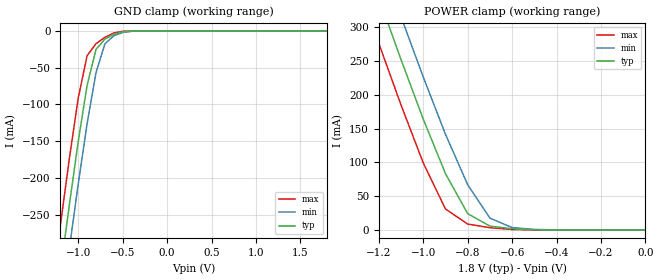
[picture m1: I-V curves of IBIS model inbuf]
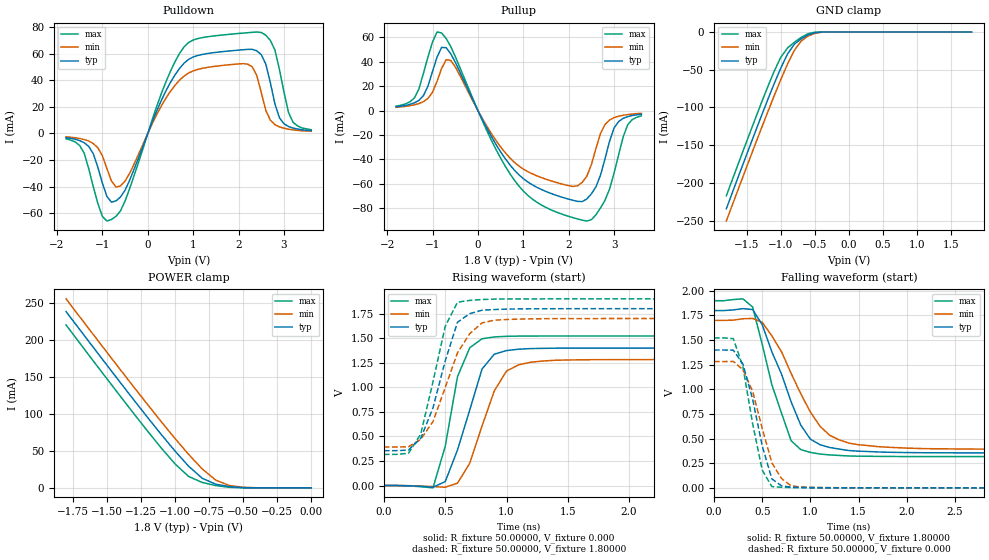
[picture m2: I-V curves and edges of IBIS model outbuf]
| IBIS file ics651_1p8.ibs created by s2ibis2 version 1.2
| North Carolina State University Electronics Research Laboratory  1995
[IBIS ver]   3.2
[File name]   ics651_1p8.ibs
[File Rev]   1.0
[Date]   March 22, 2007
[Source]   IDT
[Notes]   1. Temp typ=25C, min=+85C, max=-40C 2. Ramp rates based on 50
   ohm load
[Disclaimer] READ THESE TERMS AND CONDITIONS CAREFULLY BEFORE USING THIS
   IBIS MODEL. BY USING THIS IBIS MODEL, YOU ARE ACCEPTING AND
   AGREEING TO THESE TERMS AND CONDITIONS OF USE. Integrated
   Device Technology, Inc. ("IDT") hereby grants the user of this
   IBIS model ("User") a non-exclusive, nontransferable license
   to use this IBIS model under the following terms: The User is
   granted this license only to use the IBIS model for
   demonstration purposes only and is not granted rights to sell,
   copy (except as needed to run the IBIS model), rent, lease or
   sub-license (except for demonstration) the IBIS model in whole
   or in part, or in modified form to anyone. The User may modify
   the IBIS model to suit its specific applications, but rights
   to derivative works and such modifications shall belong to
   IDT. THIS IBIS MODEL IS PROVIDED ON AN AS IS" BASIS AND IDT
   MAKES ABSOLUTELY NO WARRANTY WITH RESPECT TO THE INFORMATION
   CONTAINED HEREIN. IDT DISCLAIMS AND USER WAIVES ALL
   WARRANTIES, EXPRESS AND IMPLIED, INCLUDING WARRANTIES OF
   MERCHANTABILITY AND FITNESS FOR A PARTICULAR PURPOSE. THE
   ENTIRE RISK AS TO QUALITY AND PERFORMANCE IS WITH THE USER
   ACCORDINGLY, IN NO EVENT SHALL IDT BE LIABLE FOR ANY DIRECT OR
   INDIRECT DAMAGES, WHETHER IN CONTRACT OR TORT, INCLUDING ANY
   LOST PROFITS OR OTHER INCIDENTAL, CONSEQUENTIAL, EXEMPLARY, OR
   PUNITIVE DAMAGES ARISING OUT OF THE USE OR APPLICATION OF THE
   IBIS MODEL, WHETHER OR NOT IDT HAD NOTICE OF SUCH DAMAGES. IDT
   reserves the right to make changes without notice to any
   product herein to improve reliability, function, or design.
   IDT does not convey any license under patent rights or any
   other intellectual property rights, including those of third
   parties. IDT is not obligated to provide maintenance or
   support for the licensed IBIS model.
   **************************************** This model is for
   ICS651 IDT Clock ****************************************
[Copyright]   Copyright 2007, Integrated Device Technology, Inc. All rights
   reserved.
|   Component ICS651
[Component]   ICS651
[Manufacturer]   Integrated Device Technology Inc.
[Package]
| variable   typ   min   max
R_pkg   40.00000m   35.00000m   45.00000m
L_pkg   1.65000nH   1.35000nH   1.95000nH
C_pkg   0.24000pF   0.14000pF   0.34000pF
[Pin]  signal_name   model_name   R_pin   L_pin   C_pin
1   ICLK   inbuf
2   Q1   outbuf
3   Q2   outbuf
4   Q3   outbuf
5   Q4   outbuf
6   GND   GND
7   VDD   POWER
8   OE   inbuf
| Models and submodels in the file (2): inbuf (Input), outbuf (3-state)
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| in   in   dummy
| oe   oe   dummy
|   Model inbuf
[Model]   inbuf
Model_type   Input
Vinl =  0.63000V
Vinh =  1.17000V
C_comp   5.50000pF   5.00000pF   6.00000pF
[Temperature Range]   25.00000   85.00000   -40.00000
[Voltage Range]   1.80000V   1.70000V   1.90000V
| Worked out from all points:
|   GND clamp passes 1 mA (typ) near -0.50 V on its own axis
|   POWER clamp passes 1 mA (typ) near -0.55 V on its own axis
[GND_clamp]
| voltage   I(typ)   I(min)   I(max)
-1.8V     -898.9mA   -957.2mA   -837.5mA
-1.3V     -420.5mA   -480.4mA   -357mA
-1.2V     -327.6mA   -387.6mA   -264mA
-1.1V     -237mA     -296.6mA   -174mA
-1V       -150.5mA   -208.5mA   -91.29mA
-900mV    -73.81mA   -126.1mA   -33.43mA
-800mV    -24.96mA   -56.58mA   -17.15mA
-700mV    -10.96mA   -17.4mA    -8.598mA
-600mV    -4.471mA   -6.338mA   -2.511mA
-500mV    -925.8uA   -1.904mA   -242.1uA
-400mV    -81.45uA   -291.4uA   -13.93uA
1.8V      1.081nA    848.9nA    -1.089uA
[POWER_clamp]
| voltage   I(typ)   I(min)   I(max)
-1.8V     917.2mA    979.2mA    852mA
-1.3V     437.3mA    500.8mA    369.9mA
-1.2V     343.8mA    407.4mA    276.2mA
-1.1V     252.2mA    315.6mA    185mA
-1V       164.1mA    226.4mA    99.28mA
-900mV    83.43mA    141.7mA    31.04mA
-800mV    24.16mA    66.96mA    8.749mA
-700mV    5.751mA    17.53mA    3.41mA
-600mV    1.751mA    3.532mA    720.7uA
-500mV    298.4uA    782.1uA    64.85uA
-400mV    30.44uA    115.8uA    7.502uA
0V        1.081nA    29.2nA     102.5pA
|   Model outbuf
[Model]   outbuf
Model_type   3-state
Polarity   Non-Inverting
Enable   Active-Low
Vmeas =  0.90000V
Rref = 50.00000
Vref =  0.000V
C_comp   5.50000pF   5.00000pF   6.00000pF
[Temperature Range]   25.00000   85.00000   -40.00000
[Voltage Range]   1.80000V   1.70000V   1.90000V
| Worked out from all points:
|   slope of the pulldown table from 0 to 0.27 V, typ, clamps not added: 11.9 ohm
|   slope of the pullup table from 0 to 0.27 V, typ, clamps not added: 13.8 ohm
|   GND clamp passes 1 mA (typ) near -0.50 V on its own axis
|   POWER clamp passes 1 mA (typ) near -0.55 V on its own axis
|   rising waveform, R_fixture 50.00000, V_fixture 0.000: 20-80 % time 210ps typ, 223ps min, 160ps max; typ from 0 V to 1.4 V
|   rising waveform, R_fixture 50.00000, V_fixture 1.80000: 20-80 % time 209ps typ, 244ps min, 173ps max; typ from 0.355 V to 1.8 V
|   falling waveform, R_fixture 50.00000, V_fixture 1.80000: 20-80 % time 344ps typ, 415ps min, 278ps max; typ from 1.8 V to 0.355 V
|   falling waveform, R_fixture 50.00000, V_fixture 0.000: 20-80 % time 205ps typ, 219ps min, 172ps max; typ from 1.4 V to 0 V
[Pulldown]
| voltage   I(typ)   I(min)   I(max)
-1.8V     -3.2mA     -2.5mA     -4mA
-1.3V     -9.8mA     -5.7mA     -26.65mA
-1V       -37.38mA   -16.83mA   -62.43mA
-800mV    -51.67mA   -35.82mA   -64.64mA
-500mV    -42.63mA   -35.75mA   -50.75mA
300mV     24.94mA    20.82mA    30.1mA
800mV     52.83mA    43.14mA    65.09mA
2.4V      62.08mA    43.6mA     76.17mA
2.6V      52.01mA    17.3mA     73.75mA
2.9V      11.67mA    4.9mA      48mA
3.2V      4mA        2.7mA      8.35mA
3.6V      2.1mA      1.7mA      2.8mA
[Pullup]
| voltage   I(typ)   I(min)   I(max)
-1.8V     3.1mA      2.6mA      3.6mA
-1.4V     6.3mA      4.7mA      10.3mA
-1.2V     12.23mA    7.3mA      30.55mA
-800mV    51.83mA    34.56mA    63.73mA
-600mV    46.63mA    41.18mA    52.66mA
900mV     -52.67mA   -45.5mA    -61.86mA
2.1V      -73.75mA   -62.33mA   -88mA
2.4V      -72.54mA   -53.8mA    -90.69mA
2.8V      -39.53mA   -11.4mA    -73.56mA
3V        -14.21mA   -5.8mA     -51.09mA
3.3V      -5mA       -3.3mA     -11.6mA
3.6V      -3mA       -2.3mA     -4.3mA
[GND_clamp]
| voltage   I(typ)   I(min)   I(max)
-1.8V     -234.3mA   -250.6mA   -217.2mA
-1.3V     -114.7mA   -131.2mA   -97.35mA
-1.1V     -69.05mA   -85.13mA   -52.51mA
-1V       -47.67mA   -63.05mA   -33.38mA
-900mV    -28.89mA   -42.27mA   -21.03mA
-800mV    -16.04mA   -24.21mA   -13.46mA
-700mV    -8.94mA    -11.82mA   -7.05mA
-600mV    -3.886mA   -5.387mA   -2.229mA
-500mV    -872.3uA   -1.753mA   -231uA
-400mV    -76.24uA   -282.3uA   -7.635uA
1.8V      1.081nA    92.98nA    85.97pA
[POWER_clamp]
| voltage   I(typ)   I(min)   I(max)
-1.8V     238.4mA    255.6mA    220.3mA
-1.4V     142mA      159.4mA    123.5mA
-1.2V     94.87mA    112.3mA    76.35mA
-1V       49.75mA    66.73mA    32.37mA
-900mV    29.23mA    45.17mA    15.35mA
-800mV    12.89mA    25.5mA     7.266mA
-700mV    4.877mA    10.33mA    3.05mA
-600mV    1.627mA    3.084mA    683.2uA
-500mV    287.7uA    748.1uA    58.05uA
-400mV    26.31uA    111.6uA    2.376uA
0V        1.081nA    29.2nA     102.5pA
[Ramp]
| variable   typ   min   max
dV/dt_r   0.83940/0.17056n   0.76920/0.21229n   0.91320/0.13298n
dV/dt_f   0.86700/0.31530n   0.78468/0.40017n   0.94968/0.24247n
R_load = 50.00000
[Rising Waveform]
R_fixture = 50.00000
V_fixture = 0.000
V_fixture_min = 0.000
V_fixture_max = 0.000
| time   V(typ)   V(min)   V(max)
0s        0V         0V         0V
400ps     -16.88mV   -10.28mV   -23.47mV
500ps     40.1mV     -17.2mV    399.2mV
600ps     362mV      23.92mV    1.108V
700ps     769.4mV    227.1mV    1.403V
800ps     1.185V     604.8mV    1.494V
900ps     1.337V     962.4mV    1.512V
1ns       1.374V     1.166V     1.519V
1.2ns     1.394V     1.256V     1.522V
5ns       1.399V     1.282V     1.522V
[Rising Waveform]
R_fixture = 50.00000
V_fixture = 1.80000
V_fixture_min = 1.70000
V_fixture_max = 1.90000
| time   V(typ)   V(min)   V(max)
0s        354.9mV    392.2mV    317.2mV
200ps     361mV      394.5mV    328.1mV
300ps     479.6mV    470.5mV    522.9mV
400ps     791mV      651.1mV    1.056V
500ps     1.269V     998.2mV    1.621V
600ps     1.662V     1.351V     1.866V
700ps     1.75V      1.546V     1.885V
800ps     1.784V     1.655V     1.893V
900ps     1.792V     1.683V     1.897V
5ns       1.8V       1.7V       1.9V
[Falling Waveform]
R_fixture = 50.00000
V_fixture = 1.80000
V_fixture_min = 1.70000
V_fixture_max = 1.90000
| time   V(typ)   V(min)   V(max)
0s        1.8V       1.7V       1.9V
300ps     1.819V     1.716V     1.918V
400ps     1.81V      1.72V      1.836V
600ps     1.38V      1.542V     1.047V
800ps     873.3mV    1.161V     478.7mV
900ps     636.9mV    955.5mV    388.6mV
1ns       494.3mV    769.4mV    359.6mV
1.2ns     409.6mV    533.9mV    334.5mV
1.5ns     372.1mV    437.7mV    321.5mV
5ns       355mV      392.2mV    317.2mV
[Falling Waveform]
R_fixture = 50.00000
V_fixture = 0.000
V_fixture_min = 0.000
V_fixture_max = 0.000
| time   V(typ)   V(min)   V(max)
0s        1.399V     1.282V     1.522V
200ps     1.398V     1.283V     1.514V
300ps     1.256V     1.199V     1.227V
400ps     900.7mV    981.4mV    653.1mV
500ps     426mV      604.1mV    180.2mV
600ps     90.88mV    253.4mV    12.54mV
700ps     20.48mV    94.8mV     6.165mV
800ps     6.904mV    20.68mV    2.93mV
900ps     4.207mV    7.947mV    1.671mV
5ns       9.176uV    1.534uV    4.225uV
